FUNCTION "FC_Gest_CalendarioV2.1" : VOID
TITLE =
//Nome     : Gestione Calendario
//Codice   : n.a.
//Famiglia : n.a.
//PLC      : S7-300/400
//HMI      : Tia Portal
//Release  : 02.01.00
//Data     : 2021.12.20
//Autore   : Coletta Simone
//Nemesis  :
{ S7_language := '9(1) Inglese (Stati Uniti)  05.10.2016  15:47:09' }
NAME : ColettaS
VERSION : 2.1


VAR_INPUT
  cDB : BLOCK_DB ;
  CurrentDay : BYTE ;
  CurrentHour : BYTE ;
  CurrentMinute : BYTE ;
  EnHourShutDown : BOOL ;
  HourShutDown : INT ;
  MinuteShutDown : INT ;
  Week : BOOL ;	//=1 Prog Week
END_VAR
VAR_TEMP
  Manual : BOOL ;	//Manual Cycle Selection
  PB_Read : BOOL ;	//PB Read
  PB_Edit : BOOL ;	//PB Edit
  PB_Write : BOOL ;	//PB Write
  PointDay_Edited : BOOL ;
  EditingEnabled : BOOL ;
  DayPointer : INT ;
  ReadPointer : WORD ;
  WritePointer : WORD ;
  _Pointer : WORD ;
  hmiPointer : INT ;
  SAVE_AR1 : DWORD ;
  AUX : "UDT_CalendarioV2";
END_VAR
BEGIN
NETWORK
TITLE =



NETWORK
TITLE =Zero-flag for parameterization


//  U     #Enable
//   =     #Manual
NETWORK
TITLE =



NETWORK
TITLE =CARICAMENTO DB

      AUF   #cDB;

NETWORK
TITLE =Gestione Modifica



      ON    DBX   36.0;
      O     DBX   36.2;
      =     #Manual;

      U     DBX   36.4;
      U(    ;
      O(    ;
      L     DBW   16;
      L     #CurrentDay;
      ==I   ;
      )     ;
      O(    ;
      L     #CurrentDay;
      L     1;
      +I    ;
      L     DBW   16;
      ==I   ;
      )     ;
      )     ;
      =     #PB_Write;
      R     DBX   36.4;
      R     DBX   36.3;

      U     DBX   36.4;
      S     DBX   36.3;
      R     DBX   36.4;

      U     DBX   36.1;
      =     #PB_Read;
      R     DBX   36.1;

      U     #Manual;
      U     #PB_Edit;
      UN    DBX   36.7;
      UN    DBX   36.6; //antiripetizione
      S     DBX   36.7;
      S     DBX   36.6; //antiripetizione

      U     #Manual;
      U     #PB_Edit;
      U     DBX   36.7;
      UN    DBX   36.6; //antiripetizione
      R     DBX   36.7;
      S     DBX   36.6; //antiripetizione

      UN    #PB_Edit;
      R     DBX   36.6; //antiripetizione

      UN    #Manual;
      R     DBX   36.7;

      U     DBX   36.7;
      =     #EditingEnabled;

      U     DBX   36.5;
      =     #PointDay_Edited;
      R     DBX   36.5;
NETWORK
TITLE =Gestione Write

      L     DBW   16; //DayPointer
      T     #DayPointer;


      U(    ;
      L     #DayPointer; // Checking range of Day
      L     1;
      >=I   ;
      )     ;
      U(    ;
      L     #DayPointer;
      L     7;
      <=I   ;
      )     ;
      SPBNB M004;


      U     #Manual;
      U     #PB_Write;
      SPBNB M004;

//Init READ Pointer
      L     #DayPointer;
      L     1;
      -I    ;
      T     #WritePointer;
      L     16;
      *I    ;
      T     #WritePointer;
      L     54;
      +I    ;
      T     #WritePointer;

      SLD   3;
      L     P#DBX 0.0;
      +D    ;
      LAR1  ;

//Write Data To DB

      L     DBW    0;
      T     DBW [AR1,P#0.0];
      L     DBW    2;
      T     DBW [AR1,P#2.0];
      L     DBW    4;
      T     DBW [AR1,P#4.0];
      L     DBW    6;
      T     DBW [AR1,P#6.0];
      L     DBW    8;
      T     DBW [AR1,P#8.0];



M004: NOP   0;
NETWORK
TITLE =Gestione Read

      L     DBW   16; //DayPointer
      T     #DayPointer;


      U(    ;
      L     #DayPointer; // Checking range of Day
      L     1;
      >=I   ;
      )     ;
      U(    ;
      L     #DayPointer;
      L     7;
      <=I   ;
      )     ;
      SPBNB M003;

      O     #PointDay_Edited;
      O     ;
      U     #Manual;
      U(    ;
      O     #PB_Read;
      O     #PB_Write;
// O     #PB_Edit
      )     ;
      SPBNB M003;

//Init READ Pointer
      L     #DayPointer;
      L     1;
      -I    ;
      T     #ReadPointer;
      L     16;
      *I    ;
      T     #ReadPointer;
      L     54;
      +I    ;
      T     #ReadPointer;

      SLD   3;
      L     P#DBX 0.0;
      +D    ;
      LAR1  ;

//Read Data from DB
      L     DBW [AR1,P#0.0];
      T     DBW   38;
      T     DBW    0;
      L     DBW [AR1,P#2.0];
      T     DBW   40;
      T     DBW    2;
      L     DBW [AR1,P#4.0];
      T     DBW   42;
      T     DBW    4;
      L     DBW [AR1,P#6.0];
      T     DBW   44;
      T     DBW    6;
      L     DBW [AR1,P#8.0];
      T     DBW   46;
      T     DBW    8;



M003: NOP   0;
NETWORK
TITLE =



NETWORK
TITLE =Azzeramento Area Actual Day se CurrentDay == 0

      L     #CurrentDay;
      L     0;
      ==I   ;
      SPBNB M001;
      L     0;
      T     DBW   20; //Azzeramento Area
      T     DBW   22; //Azzeramento Area
      T     DBW   24; //Azzeramento Area
      T     DBW   26;
      T     DBW   28;
M001: NOP   0;
NETWORK
TITLE =Get Actual Day from DB

// Reset Bit di Accenzione "ON"
      R     DBX  186.0;

//Verifica Giorno

      U(    ;
      L     #CurrentDay; // Checking range of Day number
      L     1;
      >=I   ;
      )     ;
      U(    ;
      L     #CurrentDay;
      L     7;
      <=I   ;
      )     ;
      SPBNB END;

//Init Pointer
      L     #CurrentDay;
      T     DBW  182;

      L     #CurrentHour;
      T     DBW  184;


      L     #CurrentDay;
      L     1;
      -I    ;
      T     #_Pointer;
      L     16;
      *I    ;
      T     #_Pointer;
      L     54;
      +I    ;
      T     #_Pointer;

      SLD   3;
      L     P#DBX 0.0;
      +D    ;
      LAR1  ;

//Read Data DB
      L     DBW [AR1,P#0.0];
      T     DBW   20;
      T     #AUX.OraStart;
      L     DBW [AR1,P#2.0];
      T     DBW   22;
      T     #AUX.MinutiStart;
      L     DBW [AR1,P#4.0];
      T     DBW   24;
      T     #AUX.OraEnd;
      L     DBW [AR1,P#6.0];
      T     DBW   26;
      T     #AUX.MinutiEnd;
      L     DBW [AR1,P#8.0];
      T     DBW   28;
      T     #AUX.Spare01;

END:  NOP   0;

      R     DBX  186.0;
NETWORK
TITLE =//Verifica accenzione
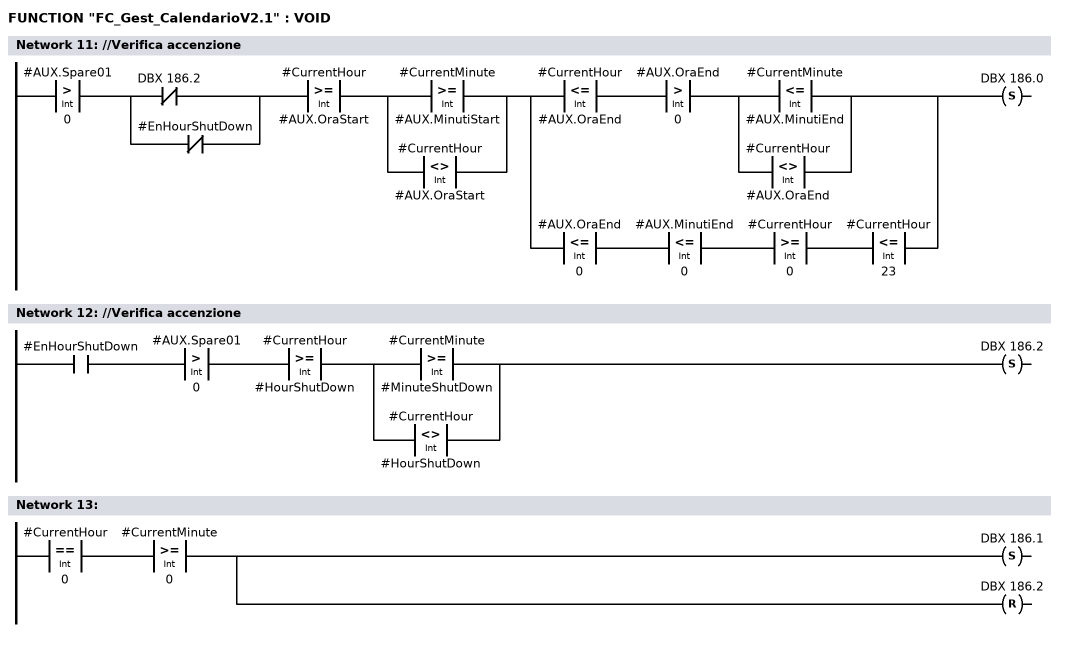
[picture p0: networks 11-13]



      U(    ;
      L     #AUX.Spare01;
      L     0;
      >I    ;
      )     ;
      U(    ;
      ON    DBX  186.2;
      ON    #EnHourShutDown;
      )     ;
      U(    ;
      L     #CurrentHour;
      L     #AUX.OraStart;
      >=I   ;
      )     ;
      U(    ;
      O(    ;
      L     #CurrentMinute;
      L     #AUX.MinutiStart;
      >=I   ;
      )     ;
      O(    ;
      L     #CurrentHour;
      L     #AUX.OraStart;
      <>I   ;
      )     ;
      )     ;
      U(    ;
      U(    ;
      L     #CurrentHour;
      L     #AUX.OraEnd;
      <=I   ;
      )     ;
      U(    ;
      L     #AUX.OraEnd;
      L     0;
      >I    ;
      )     ;
      U(    ;
      O(    ;
      L     #CurrentMinute;
      L     #AUX.MinutiEnd;
      <=I   ;
      )     ;
      O(    ;
      L     #CurrentHour;
      L     #AUX.OraEnd;
      <>I   ;
      )     ;
      )     ;
      O     ;
      U(    ;
      L     #AUX.OraEnd;
      L     0;
      <=I   ;
      )     ;
      U(    ;
      L     #AUX.MinutiEnd;
      L     0;
      <=I   ;
      )     ;
      U(    ;
      L     #CurrentHour;
      L     0;
      >=I   ;
      )     ;
      U(    ;
      L     #CurrentHour;
      L     23;
      <=I   ;
      )     ;
      )     ;
      S     DBX  186.0;
NETWORK
TITLE =//Verifica accenzione

      U     #EnHourShutDown;
      U(    ;
      L     #AUX.Spare01;
      L     0;
      >I    ;
      )     ;
      U(    ;
      L     #CurrentHour;
      L     #HourShutDown;
      >=I   ;
      )     ;
      U(    ;
      O(    ;
      L     #CurrentMinute;
      L     #MinuteShutDown;
      >=I   ;
      )     ;
      O(    ;
      L     #CurrentHour;
      L     #HourShutDown;
      <>I   ;
      )     ;
      )     ;
      S     DBX  186.2;
NETWORK
TITLE =

      U(    ;
      L     #CurrentHour;
      L     0;
      ==I   ;
      )     ;
      U(    ;
      L     #CurrentMinute;
      L     0;
      >=I   ;
      )     ;
      S     DBX  186.1;
      R     DBX  186.2;
NETWORK
TITLE =

      U     DBX  186.1;

      SPBN  End1;
//Verifica Giorno
      R     DBX  186.1;

      U(    ;
      L     #CurrentDay; // Checking range of Day number
      L     1;
      >=I   ;
      )     ;
      U(    ;
      L     #CurrentDay;
      L     7;
      <=I   ;
      )     ;
      SPBNB End1;

//Init Pointer

      U(    ;
      L     #CurrentDay; // Checking range of Day number
      L     1;
      ==I   ;
      )     ;
      SPBNB up;
      L     8;
      T     #CurrentDay;

up:   NOP   0;

      L     #CurrentDay;
      L     2;
      -I    ;
      T     #_Pointer;
      L     16;
      *I    ;
      T     #_Pointer;
      L     54;
      +I    ;
      T     #_Pointer;

      SLD   3;
      L     P#DBX 0.0;
      +D    ;
      LAR1  ;

//Write Data DB
      L     0;
      T     DBW [AR1,P#8.0];


End1: NOP   0;
END_FUNCTION

